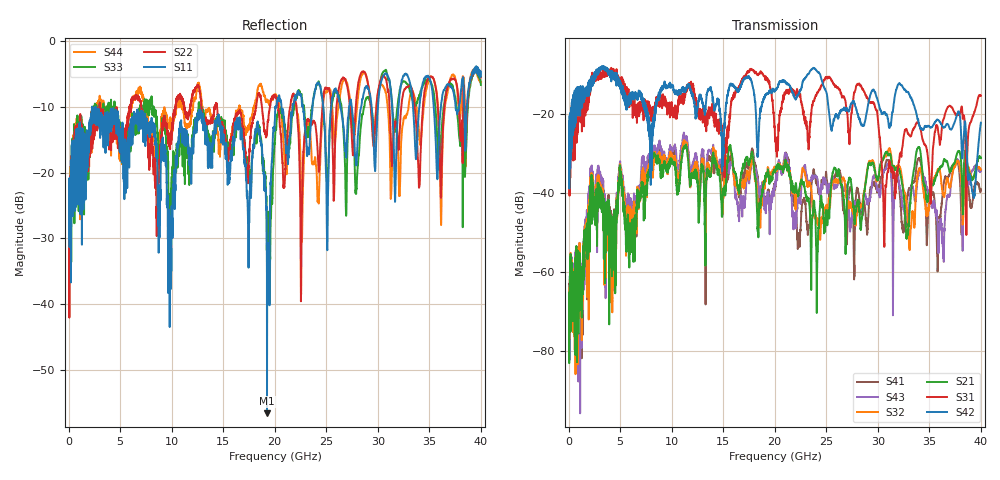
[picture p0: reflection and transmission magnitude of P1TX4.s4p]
!Agilent Technologies,N5245A,MY49151084,A.09.20.08
!Agilent N5245A: A.09.20.08
!Date: Thursday, March 01, 2012 14:06:53
!Correction: S11(Full 4 Port(1,2,3,4))
!S12(Full 4 Port(1,2,3,4))
!S13(Full 4 Port(1,2,3,4))
!S14(Full 4 Port(1,2,3,4))
!S21(Full 4 Port(1,2,3,4))
!S22(Full 4 Port(1,2,3,4))
!S23(Full 4 Port(1,2,3,4))
!S24(Full 4 Port(1,2,3,4))
!S31(Full 4 Port(1,2,3,4))
!S32(Full 4 Port(1,2,3,4))
!S33(Full 4 Port(1,2,3,4))
!S34(Full 4 Port(1,2,3,4))
!S41(Full 4 Port(1,2,3,4))
!S42(Full 4 Port(1,2,3,4))
!S43(Full 4 Port(1,2,3,4))
!S44(Full 4 Port(1,2,3,4))
!S4P File: Measurements: <S11,S12,S13,S14>,
!<S21,S22,S23,S24>,
!<S31,S32,S33,S34>,
!<S41,S42,S43,S44>:
# Hz S  dB  R 50
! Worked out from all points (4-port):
!   3996 points, 50 MHz to 40 GHz, reference 50 ohm
!   strongest paths, dB at 50 MHz, 10.04 GHz, 20.03 GHz, 30.02 GHz, 40 GHz:
!     S42: -24.8, -12.9, -14.2, -16.9, -22.3
!     S31: -26.4, -19.2, -26.5, -21.8, -15.5
!     S21: -65.7, -32.1, -34.9, -36.5, -31.2
!     S32: -64.1, -31.1, -34.2, -36.6, -34.1
!     S43: -63.6, -29.0, -37.3, -39.5, -34.5
!     S41: -63.1, -30.0, -39.3, -38.7, -39.3
!   lowest |S11| = -56.5 dB at 19.25 GHz (marker M1), VSWR 1.00, Z = 50 + j0.148 ohm
!   |S11| at or under -10 dB: start of sweep to 20.1 GHz; 20.65 GHz to 21.74 GHz (1.088 GHz wide, 5.13 % of centre); 22.74 GHz to 23.67 GHz (924.8 MHz wide, 3.99 % of centre)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
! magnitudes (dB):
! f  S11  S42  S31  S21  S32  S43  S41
! 50 MHz  -23.7  -24.8  -26.4  -65.7  -64.1  -63.6  -63.1
! 8.78 GHz  -21.9  -16.4  -17.4  -31.7  -29.8  -27.0  -29.0
! 19.25 GHz  -56.5  -15.0  -11.1  -36.0  -35.0  -41.3  -42.3
! 20.38 GHz  -8.9  -12.6  -23.6  -32.8  -33.2  -32.9  -32.2
! 28.26 GHz  -11.0  -21.8  -12.8  -46.6  -43.8  -44.6  -42.5
! 30.65 GHz  -5.1  -19.8  -51.1  -30.5  -30.9  -34.3  -34.1
! 40 GHz  -5.4  -22.3  -15.5  -31.2  -34.1  -34.5  -39.3
